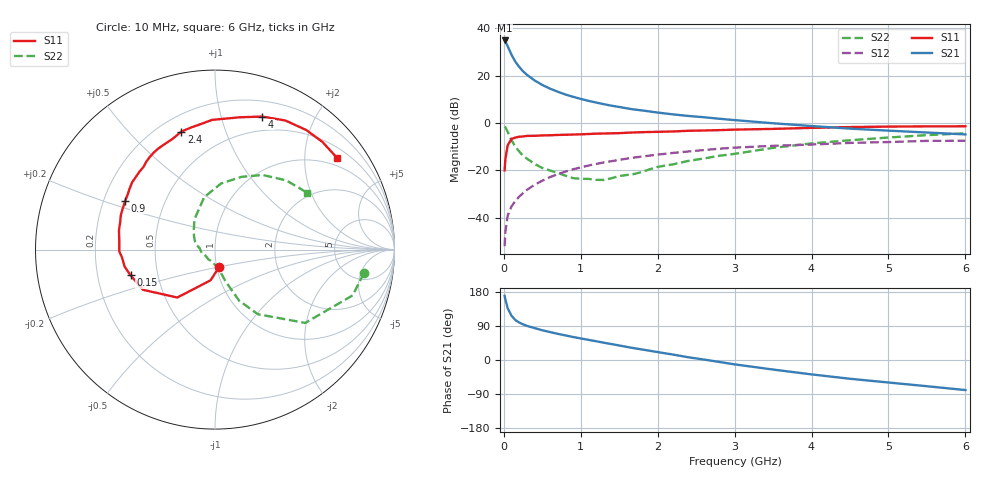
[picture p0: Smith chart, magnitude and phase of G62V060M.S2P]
! SIEMENS Small Signal Semiconductors
! BFG193
! Si NPN RF Bipolar Junction Transistor in SOT223
! VCE = 2 V  IC = 60 mA
! Common Emitter S-Parameters:  August  1996
# GHz  S  MA  R  50
!  f  S11  S21  S12  S22
! GHz  MAG  ANG  MAG  ANG  MAG  ANG  MAG  ANG
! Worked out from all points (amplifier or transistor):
!   36 points, 10 MHz to 6 GHz, reference 50 ohm
!   highest |S21| = 34.9 dB at 10 MHz (marker M1)
!   |S21| within 3 dB of that: start of sweep to 57.64 MHz
!   unconditionally stable (mu >= 1): start of sweep to 10.65 MHz; 284.3 MHz to 2.548 GHz
!   at 250 MHz: K = 0.99, MSG = 25.7 dB, |S12| = -29.6 dB
!   at 1.4 GHz: K = 1.07, MAG = 10.1 dB, |S12| = -16.1 dB
!   at 6 GHz: K = 0.95, MSG = 1.3 dB, |S12| = -7.5 dB
!   S11 on the Smith chart (normalised r, x): 10 MHz: 1.03, -0.20; 150 MHz: 0.35, -0.13; 900 MHz: 0.29, +0.23; 2.4 GHz: 0.29, +0.71; 4 GHz: 0.35, +1.36; 6 GHz: 0.76, +2.81
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0.01  0.0994 -76.7  55.27 169.3  0.0025 82.9  0.8399 -9.0
0.02  0.1727 -98.1  52.52 159.8  0.005 76.6  0.8084 -18.4
0.05  0.3398 -128.2  41.69 136.6  0.0111 67.3  0.6477 -39.1
0.1  0.4592 -150.8  27.53 116.7  0.0173 65.6  0.4323 -56.4
0.15  0.492 -163.1  19.63 105.3  0.0225 65.0  0.315 -64.7
0.2  0.5127 -169.4  15.28 98.9  0.0279 67.5  0.2504 -67.3
0.25  0.5192 -174.9  12.34 94.0  0.033 67.6  0.2024 -70.2
0.3  0.5333 -179.0  10.41 90.1  0.0386 69.1  0.1762 -72.3
0.4  0.5353 175.0  7.902 84.2  0.0496 69.1  0.1365 -75.4
0.5  0.5458 168.6  6.338 78.5  0.0603 68.1  0.1121 -77.8
0.6  0.5498 164.0  5.31 73.7  0.0719 67.1  0.0991 -82.0
0.7  0.5584 160.0  4.569 69.1  0.0828 65.5  0.0881 -88.4
0.9  0.5696 151.4  3.572 60.7  0.1051 61.5  0.0684 -101.9
1.1  0.5846 144.5  2.93 53.2  0.126 57.8  0.0659 -123.3
1.6  0.6219 127.9  2.033 34.5  0.1767 46.4  0.0797 -174.0
2.2  0.6613 110.8  1.517 14.3  0.2331 32.2  0.1336 150.1
2.4  0.6839 105.9  1.406 7.1  0.2502 27.9  0.1583 138.8
3.5  0.7497 79.5  0.986 -25.2  0.3287 0.0  0.298 101.7
4  0.7869 70.4  0.861 -38.0  0.351 -9.9  0.3701 84.7
4.5  0.8192 61.4  0.759 -49.5  0.3794 -20.1  0.4312 70.0
5.5  0.8474 45.1  0.628 -69.2  0.4189 -43.4  0.5538 44.1
6  0.8507 36.9  0.573 -79.3  0.4211 -56.6  0.6042 31.6
